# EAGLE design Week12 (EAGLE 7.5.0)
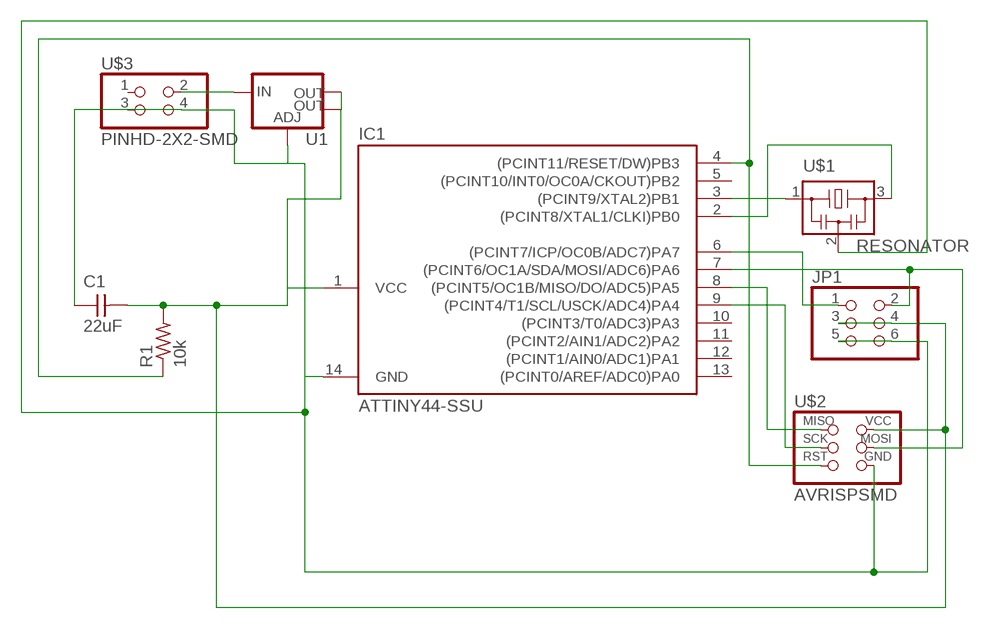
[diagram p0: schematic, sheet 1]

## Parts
C1  22uF  CAP-UNPOLARIZEDFAB  [C1206FAB]
IC1  ATTINY44-SSU  [SOIC14]
JP1  PINHD-2X3-SMD  [2X03SMD]
R1  10k  RES-US1206FAB  [R1206FAB]
U1  V_REG_LM1117SOT223  [SOT223]
U$1  RESONATOR  [EFOBM]
U$2  AVRISPSMD  [2X03SMD]
U$3  PINHD-2X2-SMD  [2X02SMD]

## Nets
N$1: U1.3(IN) U$3.2
N$3: C1.1 IC1.14(GND) JP1.5 JP1.6 U1.1(ADJ) U$1.2 U$2.6(GND) U$3.3 U$3.4
N$6: IC1.4((PCINT11/RESET/DW)PB3) R1.1 U$2.5(RST)
N$7: IC1.3((PCINT9/XTAL2)PB1) U$1.1
N$8: IC1.2((PCINT8/XTAL1/CLKI)PB0) U$1.3
N$11: IC1.8((PCINT5/OC1B/MISO/DO/ADC5)PA5) U$2.1(MISO)
N$12: IC1.9((PCINT4/T1/SCL/USCK/ADC4)PA4) U$2.3(SCK)
N$13: IC1.7((PCINT6/OC1A/SDA/MOSI/ADC6)PA6) JP1.2 U$2.4(MOSI)
N$14: IC1.6((PCINT7/ICP/OC0B/ADC7)PA7) JP1.1
N$15: C1.2 IC1.1(VCC) JP1.3 JP1.4 R1.2 U1.2(OUT) U1.4(OUT) U$2.2(VCC)
Unconnected: IC1.5((PCINT10/INT0/OC0A/CKOUT)PB2) IC1.10((PCINT3/T0/ADC3)PA3) IC1.11((PCINT2/AIN1/ADC2)PA2) IC1.12((PCINT1/AIN0/ADC1)PA1) IC1.13((PCINT0/AREF/ADC0)PA0) U$3.1

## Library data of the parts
C1 = fab:CAP-UNPOLARIZED
IC1 = fab:ATTINY44
JP1 = fab:PINHD-2X3-SMD: PIN HEADER
R1 = fab:RES-US: Resistor (US Symbol)
U1 = fab:V_REG_LM1117: Voltage Regulator LM1117 Standard adjustable voltage regulator but in SMD form. Spark Fun Electronics SKU : COM-00595; PROD_ID: VREG-08170
U$1 = fab:RESONATOR
U$2 = fab:AVRISP
U$3 = fab:PINHD-2X2-SMD

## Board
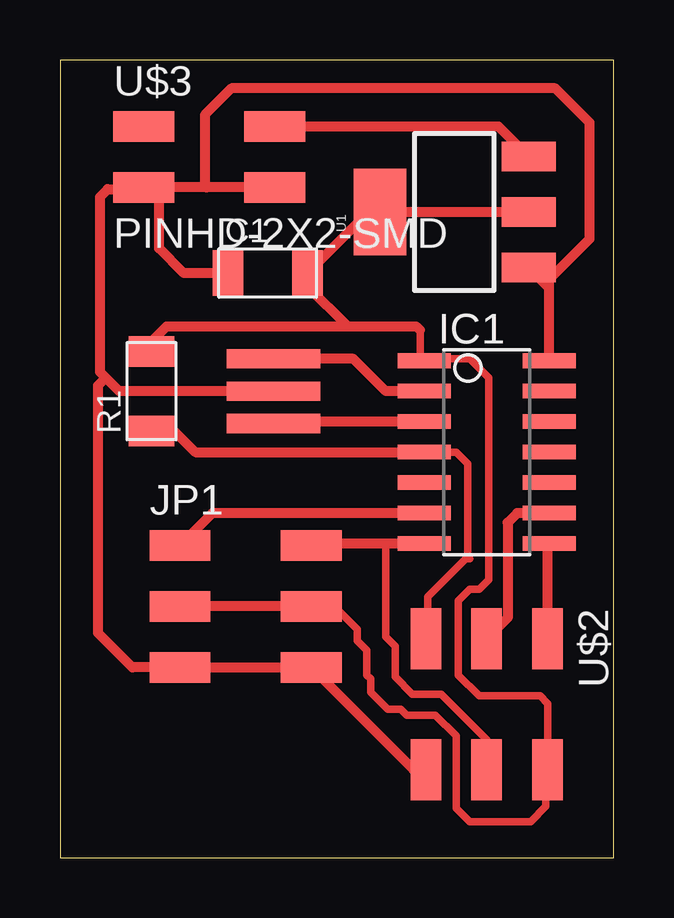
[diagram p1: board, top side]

Size 23.08 x 33.25 mm. Coordinates in mm from the lower left corner, seen from the top.
Outline: 0,0 23.08,0 23.08,33.25 0,33.25 0,0
Copper layers (1*16): Top 0.035mm / dielectric 1.5mm / Bottom 0.035mm
Design rules "default": minimum track width 10mil, minimum drill 24mil, track to track 8mil, track to pad 8mil, pad to pad 8mil, via to via 8mil, smd to smd 8mil, copper to edge 40mil, drill to drill 8mil, minimum pad ring 10mil, minimum via ring 8mil, stop-mask expansion 4mil, vias tented up to drill 0mil, thermal gap 10mil

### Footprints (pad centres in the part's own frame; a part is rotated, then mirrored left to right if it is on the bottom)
C1206FAB = smd 1.27 x 1.905: 1 -1.651,0; 2 1.651,0
SOIC14 = smd 0.61 x 2.21: 1 -3.81,-2.603; 2 -2.54,-2.603; 3 -1.27,-2.603; 4 0,-2.603; 5 1.27,-2.603; 6 2.54,-2.603; 7 3.81,-2.603; 8 3.81,2.603; 9 2.54,2.603; 10 1.27,2.603; 11 0,2.603; 12 -1.27,2.603; 13 -2.54,2.603; 14 -3.81,2.603
2X03SMD = smd 2.54 x 1.27: 1 -2.54,2.54; 2 2.92,2.54; 3 -2.54,0; 4 2.92,0; 5 -2.54,-2.54; 6 2.92,-2.54
R1206FAB = smd 1.27 x 1.905: 1 -1.651,0; 2 1.651,0
SOT223 = smd 1.219 x 2.235: 1 -2.311,-3.099; 2 0,-3.099; 3 2.311,-3.099 | smd 3.6 x 2.2: 4 0,3.099
EFOBM = smd 0.8 x 3.9: 1 -1.35,0; 2 0,0; 3 1.35,0
2X02SMD = smd 2.54 x 1.27: 1 -2.54,1.27; 2 2.92,1.27; 3 -2.54,-1.27; 4 2.92,-1.27

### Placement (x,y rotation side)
C1  8.65,24.37 0 top
IC1  17.78,16.91 270 top
JP1  7.54,10.48 0 top
R1  3.81,19.45 90 top
U1  16.43,26.91 90 top
U$1  8.89,19.45 90 top
U$2  17.78,6.59 270 top
U$3  6.03,29.21 0 top

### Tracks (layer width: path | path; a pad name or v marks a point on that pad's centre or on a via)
N$1
  Top 0.406: U$3.2 18.27,30.48 U1.3
N$3
  Top 0.406: 8.95,28.18 U$3.4 6.11,27.94 | 6.11,27.94 4.05,27.94 | 4.05,27.94 U$3.3 3.41,27.86 1.98,27.86 1.67,27.54 1.67,20.24 1.91,20 | C1.1 5.16,24.37 4.13,25.4 4.13,27.86 4.05,27.94 | U$1.2 2.46,19.45 1.91,20 | 1.91,20 1.59,19.68 1.59,9.37 3.02,7.94 JP1.5 JP1.6 14.73,3.67 U$2.6 | U1.1 20.38,23.74 IC1.14 20.38,24.11 22.07,25.8 22.07,30.64 20.64,32.07 7.14,32.07 6.03,30.96 6.03,28.02 6.11,27.94
N$6
  Top 0.305: IC1.4 16.51,16.91 16.99,16.43 16.99,12.54 17.07,12.46 16.91,12.46 15.32,10.87 15.32,9.21 U$2.5
  Top 0.406: R1.1 4.75,17.8 5.64,16.91 IC1.4
N$7
  Top 0.406: IC1.3 8.97,18.18 U$1.1
N$8
  Top 0.406: IC1.2 13.57,19.45 12.22,20.8 U$1.3
N$11
  Top 0.406: U$2.1 20.32,13.03 IC1.8
N$12
  Top 0.406: IC1.9 19.05,14.37 18.65,13.97 18.65,10 U$2.3
N$13
  Top 0.305: U$2.4 17.78,4.92 15.88,6.83 14.68,6.83 13.97,7.54 13.97,8.81 13.57,9.21 13.57,12.94 13.41,13.1
  Top 0.406: IC1.7 13.41,13.1 10.54,13.1 JP1.2
N$14
  Top 0.406: IC1.6 6.35,14.37 JP1.1
N$15
  Top 0.305: 15,21.99 15,20.89 IC1.1 15.26,20.8 17.07,20.8 17.86,20 17.86,11.59 17.46,11.19 17.07,11.19 16.59,10.72 16.59,7.62 17.46,6.75 20,6.75 20.32,6.43 U$2.2 20.24,3.59 20.24,2.14 19.61,1.51 17.07,1.51 16.51,2.06 16.51,5.08 15.64,5.95 14.45,5.95 14.21,6.19 13.65,6.19 12.94,6.91 12.94,7.46 12.78,7.62 12.78,8.65 12.38,9.05 12.38,9.53 11.43,10.48 JP1.4
  Top 0.406: JP1.4 JP1.3 | R1.2 3.81,21.51 4.45,22.15 11.99,22.15 | 11.99,22.15 14.84,22.15 15,21.99 | U1.2 U1.4 12.84,26.91 C1.2 10.3,23.83 11.99,22.15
